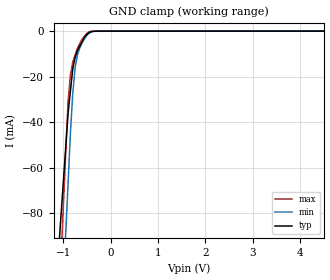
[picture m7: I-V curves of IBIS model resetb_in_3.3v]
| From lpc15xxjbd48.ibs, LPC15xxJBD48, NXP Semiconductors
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[Model] resetb_in_3.3v
Model_type Input
Vinl = 990.000mV
Vinh = 2.31000V
C_comp 1.24000pF 1.24000pF 1.24000pF
| variable typ   min   max
[Voltage Range] 3.30000V 3.00000V 3.60000V
[POWER Clamp Reference] 3.30000V 3.00000V 3.60000V
[GND Clamp Reference] 0.00000V 0.00000V 0.00000V
[Temperature Range]   25   85   -40
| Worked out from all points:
|   GND clamp passes 1 mA (typ) near -0.48 V on its own axis
[GND Clamp]
-3.3V     -761.5mA   -1.137A    -1.144A
-900mV    -36.28mA   -67.19mA   -31.14mA
-850mV    -26.36mA   -44.9mA    -19.31mA
-800mV    -16.45mA   -27.39mA   -13.61mA
-750mV    -11.56mA   -16.02mA   -10.52mA
-700mV    -8.486mA   -10.27mA   -7.436mA
-650mV    -6.523mA   -7.298mA   -5.415mA
-550mV    -2.599mA   -3.391mA   -2.127mA
-450mV    -585.3uA   -882.3uA   -285.4uA
-350mV    -42.25uA   -99.66uA   -49.08uA
-175mV    -2.578uA   -23.23uA   -2.918uA
6.6V      3.637uA    17.24uA    4.196uA
[POWER Clamp]
-3.3V     0A         0A         0A
6.6V      0A         0A         0A
